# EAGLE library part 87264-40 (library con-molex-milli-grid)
RECEPTACAL
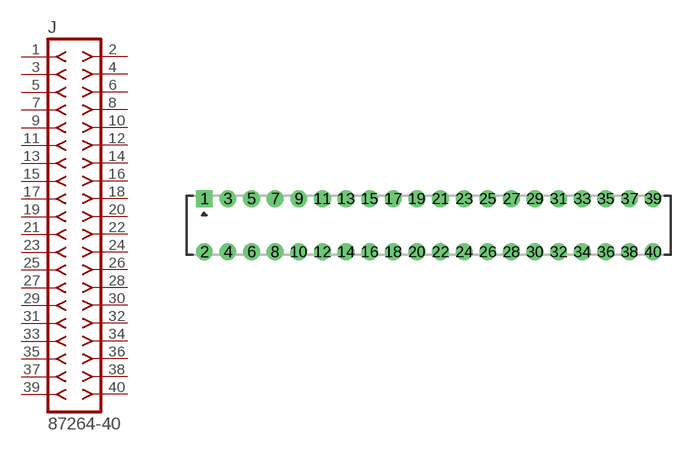
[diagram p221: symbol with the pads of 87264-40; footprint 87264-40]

Designator prefix J

## 87264-40  [87264-40]
1  1  pas
2  2  pas
3  3  pas
4  4  pas
5  5  pas
6  6  pas
7  7  pas
8  8  pas
9  9  pas
10  10  pas
11  11  pas
12  12  pas
13  13  pas
14  14  pas
15  15  pas
16  16  pas
17  17  pas
18  18  pas
19  19  pas
20  20  pas
21  21  pas
22  22  pas
23  23  pas
24  24  pas
25  25  pas
26  26  pas
27  27  pas
28  28  pas
29  29  pas
30  30  pas
31  31  pas
32  32  pas
33  33  pas
34  34  pas
35  35  pas
36  36  pas
37  37  pas
38  38  pas
39  39  pas
40  40  pas

## Footprint 87264-40 (pad centres in mm)
RECEPTACAL Dual Row, Side Entry
drill 0.914 square: 1 -19,2.25
drill 0.914: 2 -19,-2.25; 3 -17,2.25; 4 -17,-2.25; 5 -15,2.25; 6 -15,-2.25; 7 -13,2.25; 8 -13,-2.25; 9 -11,2.25; 10 -11,-2.25; 11 -9,2.25; 12 -9,-2.25; 13 -7,2.25; 14 -7,-2.25; 15 -5,2.25; 16 -5,-2.25; 17 -3,2.25; 18 -3,-2.25; 19 -1,2.25; 20 -1,-2.25; 21 1,2.25; 22 1,-2.25; 23 3,2.25; 24 3,-2.25; 25 5,2.25; 26 5,-2.25; 27 7,2.25; 28 7,-2.25; 29 9,2.25; 30 9,-2.25; 31 11,2.25; 32 11,-2.25; 33 13,2.25; 34 13,-2.25; 35 15,2.25; 36 15,-2.25; 37 17,2.25; 38 17,-2.25; 39 19,2.25; 40 19,-2.25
